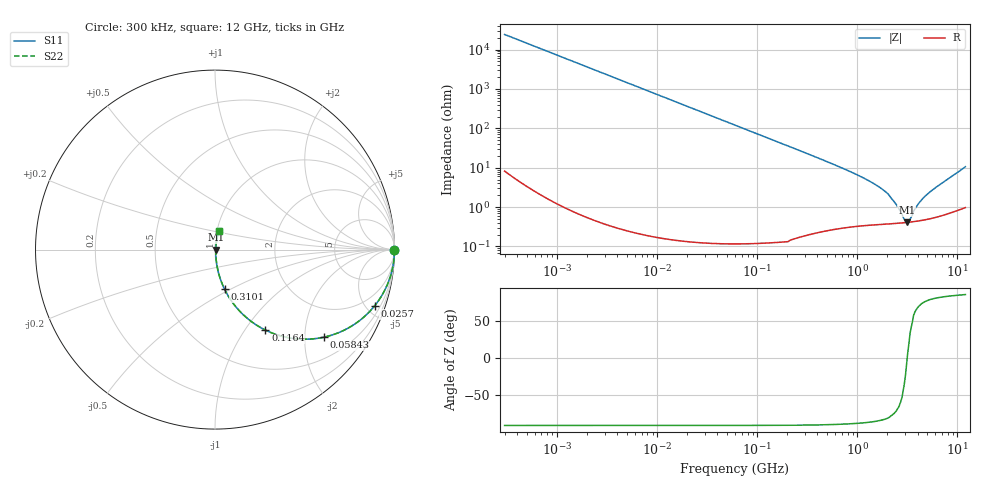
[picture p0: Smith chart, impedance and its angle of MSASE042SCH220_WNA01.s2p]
! MSASE042SCH220_WNA01  S-PARAMETER MODEL  ( General Type )
! Model Generated by TAIYO YUDEN Corporation (http://www.ty-top.com)
! Version 4.0
! TAIYO YUDEN Control No. 120810
! Copyright(c) 2007 TAIYO YUDEN CO.,LTD. All Rights Reserved.
! Product Description (link to TY-COMPAS)
! https://ds.yuden.co.jp/TYCOMPAS/or/detail?pn=MSASE042SCH220JWNA01&u=M
! Products Name : Multilayer Ceramic Capacitors
! Characteristics :
!  Capacitance : 22 pF , Rated Voltage : 16V , TCC : CH / C0H
!  Case Size : 0.4 x 0.2 / 0.016 x 0.008 [mm/inch] , Thickness : 0.2 / 0.008 [mm/inch]
!  (Conditions: Temperature = 25 degC , DC Bias Current/Voltage = 0A / 0V)
! External Node Assignments :
!  1  o---| |---o  2
! GND o---------o GND
! Frequency Range : 0.3MHz  -  12000MHz  [ 401 STEP ]
# MHz S RI R 50
! Freq[MHz].  S11 Real  S11 Imag  S21 Real  S21 Imag  S12 Real  S12 Imag  S22 Real  S22 Imag
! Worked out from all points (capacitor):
!   401 points, 300 kHz to 12 GHz, reference 50 ohm
!   read as one part in series: C = 21.9 pF near 316.3 kHz
!   lowest |Z| = 409 mohm at 3.108 GHz (marker M1)
!   series resonance near 3.148 GHz, so ESL is about 120 pH
!   S11 on the Smith chart (normalised r, x): 300 kHz: open; 25.7 MHz: 1.00, -5.67; 58.43 MHz: 1.00, -2.49; 116.4 MHz: 1.00, -1.25; 310.1 MHz: 1.00, -0.47; 12 GHz: 1.02, +0.21
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0.3  1 -0.00412  1.84e-05 0.00412  1.84e-05 0.00412  1 -0.00412
1.769972  0.9994 -0.0243  0.000594 0.0243  0.000594 0.0243  0.9994 -0.0243
10.44266  0.9798 -0.1405  0.0202 0.1405  0.0202 0.1405  0.9798 -0.1405
25.70316  0.8891 -0.3138  0.1109 0.3138  0.1109 0.3138  0.8891 -0.3138
38.24403  0.7836 -0.4115  0.2164 0.4115  0.2164 0.4115  0.7836 -0.4115
58.43137  0.6081 -0.4877  0.3919 0.4877  0.3919 0.4877  0.6081 -0.4877
60  0.5954 -0.4903  0.4046 0.4903  0.4046 0.4903  0.5954 -0.4903
82.45425  0.438 -0.4955  0.562 0.4955  0.562 0.4955  0.438 -0.4955
116.3536  0.2813 -0.4487  0.7187 0.4487  0.7187 0.4487  0.2813 -0.4487
182.544  0.1373 -0.3426  0.8627 0.3426  0.8627 0.3426  0.1373 -0.3426
310.0777  0.053 -0.2199  0.947 0.2199  0.947 0.2199  0.053 -0.2199
353.9943  0.0415 -0.1943  0.9585 0.1943  0.9585 0.1943  0.0415 -0.1943
1166.079  0.00624 -0.0535  0.9938 0.0535  0.9938 0.0535  0.00624 -0.0535
1689.663  0.00454 -0.0306  0.9955 0.0306  0.9955 0.0306  0.00454 -0.0306
2088.533  0.00409 -0.019  0.9959 0.019  0.9959 0.019  0.00409 -0.019
2448.343  0.00395 -0.0109  0.996 0.0109  0.996 0.0109  0.00395 -0.0109
2947.191  0.004 -0.00273  0.996 0.00273  0.996 0.00273  0.004 -0.00273
3107.553  0.00405 -0.000507  0.996 0.000507  0.996 0.000507  0.00405 -0.000507
3364.605  0.00414 0.00272  0.9959 -0.00272  0.9959 -0.00272  0.00414 0.00272
3944.255  0.00446 0.00982  0.9955 -0.00982  0.9955 -0.00982  0.00446 0.00982
4875.354  0.00516 0.0193  0.9948 -0.0193  0.9948 -0.0193  0.00516 0.0193
12000  0.0203 0.1025  0.9797 -0.1025  0.9797 -0.1025  0.0203 0.1025
